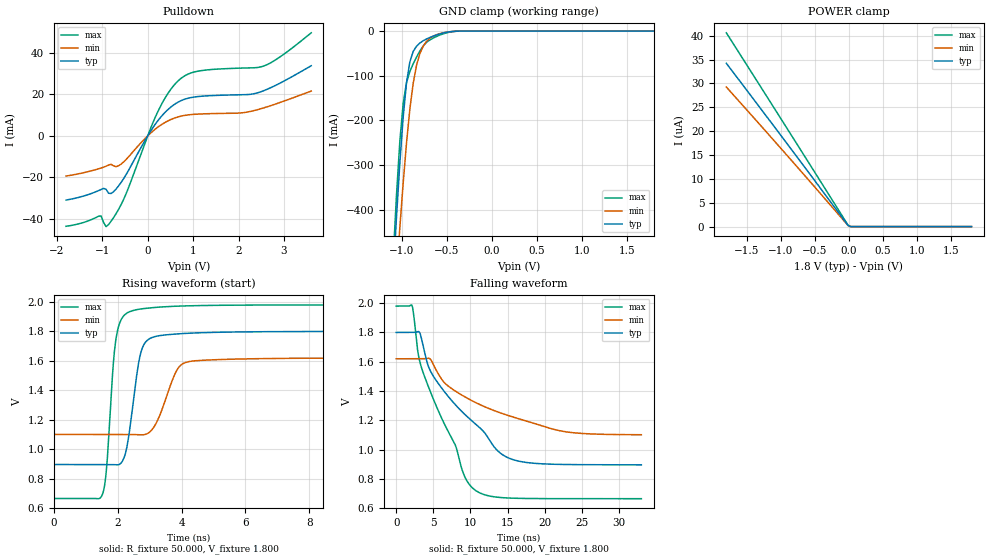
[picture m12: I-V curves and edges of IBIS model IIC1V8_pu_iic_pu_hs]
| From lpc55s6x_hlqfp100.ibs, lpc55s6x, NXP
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|   Model IIC1V8_pu_iic_pu_hs
[Model] IIC1V8_pu_iic_pu_hs
Model_type I/O_open_drain
Polarity   Non-Inverting
Enable   Active-Low
Vinl =  0.540V
Vinh =  1.260V
Vmeas =  0.900V
Cref =  0.0F
Rref =  100.000
Vref =  1.800V
C_comp   2.515pF   2.512pF   2.536pF
C_comp_pulldown   1.734pF   1.669pF   1.790pF
C_comp_power_clamp   0.457pF   0.390pF   0.548pF
[Model Spec]
Vinh   1.260V   1.134V   1.386V
Vinl   0.540V   0.486V   0.594V
Vmeas   0.900V   0.810V   0.990V
Vref   1.800V   1.620V   1.980V
Cref   0.0F   0.0F   0.0F
Rref   100.000   100.000   100.000
[Temperature Range]   25.000   0.125k   -40.000
[Voltage Range]   1.800V   1.620V   1.980V
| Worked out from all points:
|   slope of the pulldown table from 0 to 0.27 V, typ, clamps not added: 31.5 ohm
|   GND clamp passes 1 mA (typ) near -0.44 V on its own axis
|   rising waveform, R_fixture 50.000, V_fixture 1.800: 20-80 % time 347ps typ, 537ps min, 253ps max; typ from 0.895 V to 1.8 V
|   falling waveform, R_fixture 50.000, V_fixture 1.800: 20-80 % time 8.38ns typ, 11.2ns min, 5.71ns max; typ from 1.8 V to 0.896 V
[Pulldown]
|Voltage   I(typ)   I(min)   I(max)
-1.8V     -30.97mA   -19.41mA   -43.61mA
-1.03V    -25.91mA   -15.56mA   -38.59mA
-920mV    -25.75mA   -14.67mA   -43.75mA
-865mV    -27.69mA   -14.16mA   -42.79mA
-700mV    -25.69mA   -14.87mA   -37.58mA
-480mV    -18.8mA    -11.48mA   -28.03mA
235mV     7.619mA    4.356mA    12.23mA
455mV     12.83mA    7.267mA    20.76mA
730mV     16.88mA    9.427mA    27.6mA
1.17V     19mA       10.49mA    31.33mA
2.545V    21.61mA    13.36mA    33.53mA
3.6V      33.71mA    21.52mA    49.57mA
[GND_clamp]
|Voltage   I(typ)   I(min)   I(max)
-1.8V     -3.488A    -3.23A     -3.872A
-1.097V   -545.6mA   -658.5mA   -507.1mA
-1.06V    -414.6mA   -546.1mA   -365.1mA
-1.023V   -294.9mA   -439.1mA   -246mA
-986mV    -192.5mA   -339.6mA   -162mA
-949mV    -115.7mA   -250.4mA   -115.2mA
-912mV    -69.22mA   -175.3mA   -90.67mA
-838mV    -34.06mA   -77.19mA   -58.54mA
-764mV    -21.86mA   -34.13mA   -33.64mA
-653mV    -11.47mA   -11.68mA   -15.87mA
-431mV    -870uA     -906.4uA   -1.185mA
1.8V      0A         0A         0A
[POWER_clamp]
|Voltage   I(typ)   I(min)   I(max)
-1.8V     34.22uA    29.25uA    40.61uA
-864mV    16.54uA    14.2uA     19.57uA
-13mV     251.2nA    223.3nA    296.4nA
24mV      0A         0A         0A
1.8V      0A         0A         0A
[Ramp]
| variable   typ   min   max
dV/dt_r   0.543/0.347n   0.312/0.537n   0.790/0.254n
dV/dt_f   0.543/8.379n   0.311/11.175n   0.789/5.715n
R_load = 50.000
[Rising Waveform]
R_fixture= 50.000
V_fixture= 1.800
V_fixture_min= 1.620
V_fixture_max= 1.980
|time   V(typ)   V(min)   V(max)
0s        895.1mV    1.1V       664.1mV
1.507ns   895.1mV    1.1V       684.3mV
1.646ns   895.3mV    1.1V       857.9mV
1.977ns   892.5mV    1.1V       1.788V
2.28ns    1.005V     1.1V       1.924V
2.632ns   1.556V     1.097V     1.949V
2.987ns   1.749V     1.114V     1.959V
3.877ns   1.783V     1.545V     1.972V
4.445ns   1.79V      1.601V     1.975V
33ns      1.8V       1.62V      1.98V
[Falling Waveform]
R_fixture= 50.000
V_fixture= 1.800
V_fixture_min= 1.620
V_fixture_max= 1.980
|time   V(typ)   V(min)   V(max)
0s        1.8V       1.62V      1.98V
2.128ns   1.8V       1.62V      1.984V
2.935ns   1.806V     1.62V      1.662V
3.535ns   1.729V     1.62V      1.539V
5.115ns   1.492V     1.569V     1.331V
7.983ns   1.305V     1.399V     1.027V
9.238ns   1.24V      1.36V      813.4mV
10.52ns   1.181V     1.325V     726.6mV
16.18ns   924.6mV    1.215V     667mV
33ns      895.7mV    1.101V     664.3mV
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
